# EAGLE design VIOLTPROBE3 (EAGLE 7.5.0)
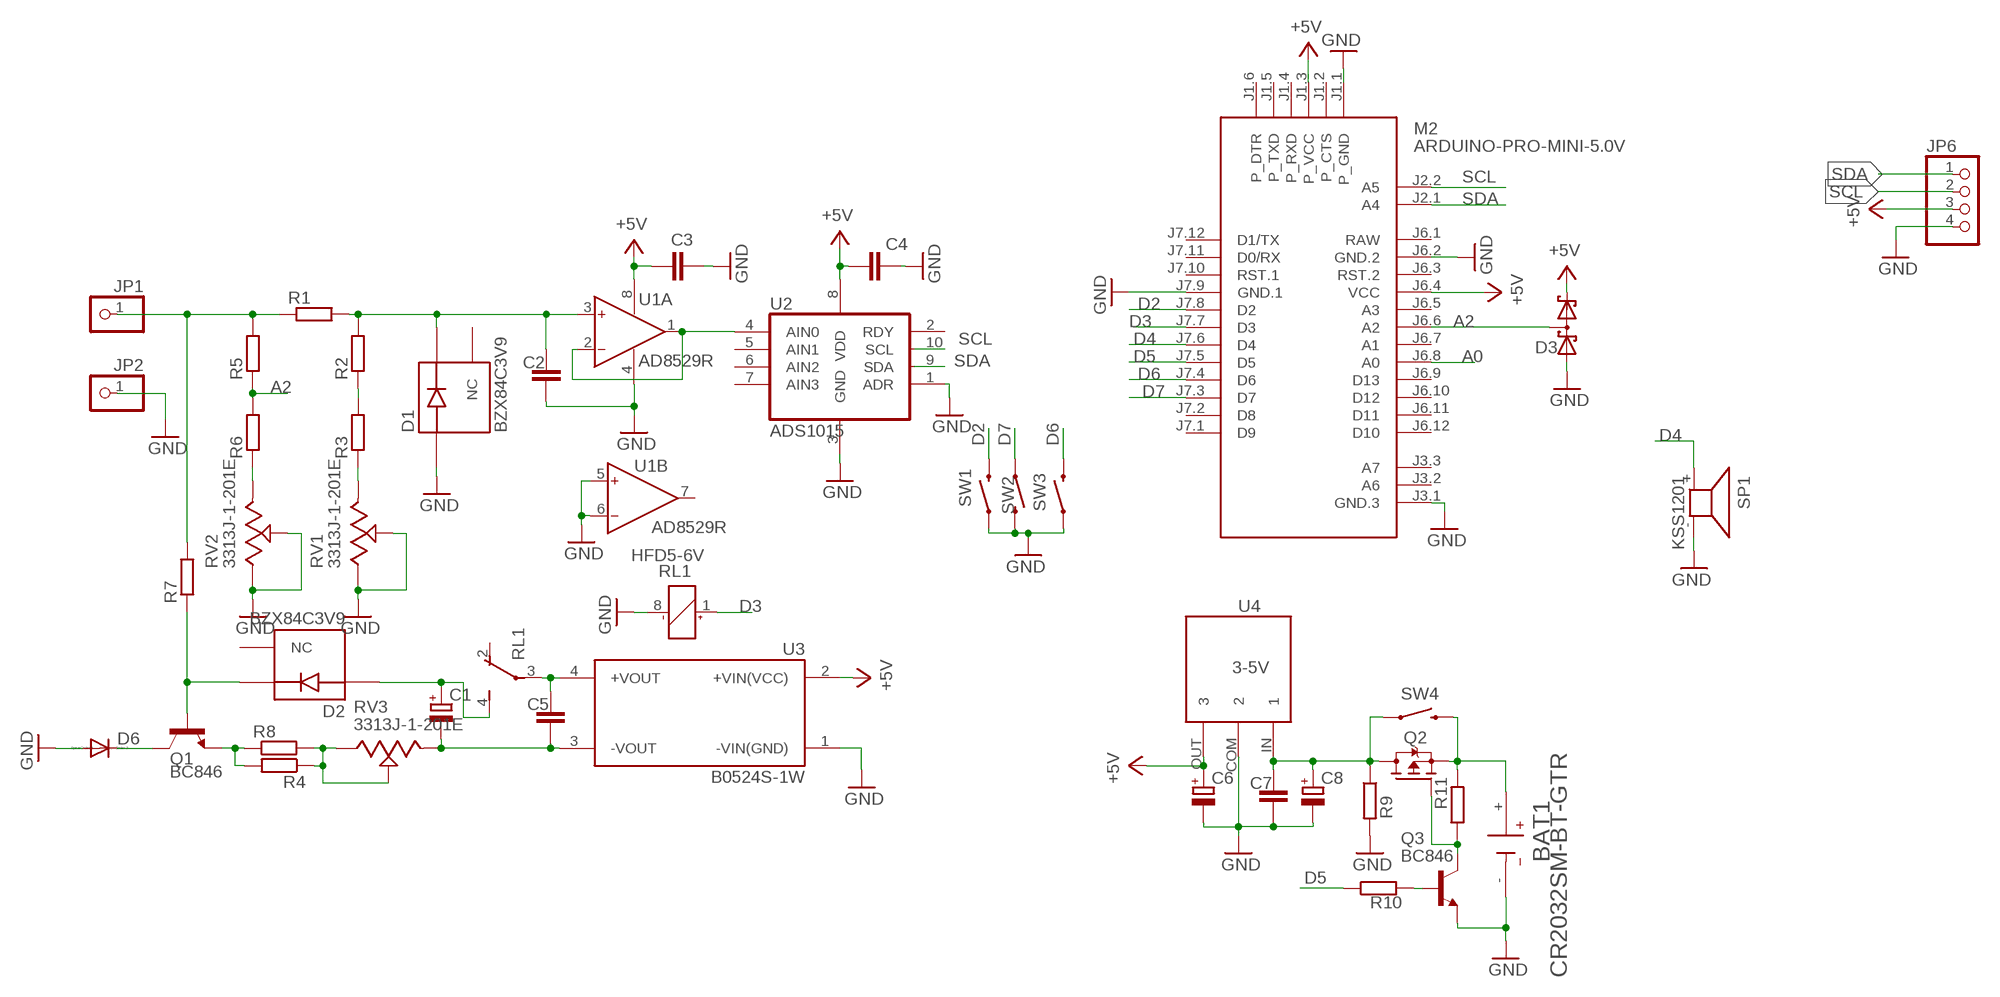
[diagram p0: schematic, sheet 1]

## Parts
BAT1  CR2032SM-BT-GTR  BU2032SM-BT-GTR  [BAT_BU2032SM-BT-GTR]
C1  CPOL-EUSMCA  [SMC_A]
C2  C-EUC0805  [C0805]
C3  C-EUC0805  [C0805]
C4  C-EUC0805  [C0805]
C5  C-EUC0805  [C0805]
C6  CPOL-EUSMCB  [SMC_B]
C7  C-EUC0805  [C0805]
C8  CPOL-EUSMCB  [SMC_B]
D1  BZX84C3V9  BZX84C15  [SOT95P237X112-3N]
D2  BZX84C3V9  BZX84C15  [SOT95P237X112-3N]
D3  BAT54S  [SOT23]
D6  CGRM4003-G  [SOD-123_MINI-SMA]
JP1  PINHD-1X1CB  [1X01-CLEANBIG]
JP2  PINHD-1X1CB  [1X01-CLEANBIG]
JP6  HEADER-1X4ROUND  [1X04_ROUND]
M2  ARDUINO-PRO-MINI-5.0V  [ARDUINO-PRO-MINI]
Q1  BC846  [SOT23]
Q2  STR2P3LLH6  [SOT23]
Q3  BC846  [SOT23]
R1  R-EU_R0603  [R0603]
R2  R-EU_R0603  [R0603]
R3  R-EU_R0603  [R0603]
R4  R-EU_R0603  [R0603]
R5  R-EU_R0603  [R0603]
R6  R-EU_R0603  [R0603]
R7  R-EU_R0603  [R0603]
R8  R-EU_R0603  [R0603]
R9  R-EU_R0603  [R0603]
R10  R-EU_R0603  [R0603]
R11  R-EU_R0603  [R0603]
RL1  HFD5-6V  G6J-2P-Y  [G6J-2P-Y]
RV1  3313J-1-201E  [TRIM_3313J-1-201E]
RV2  3313J-1-201E  [TRIM_3313J-1-201E]
RV3  3313J-1-201E  [TRIM_3313J-1-201E]
SP1  KSS1201  [KSS1201]
SW1  SWITCH-MOMENTARY-2SMD  [TACTILE-SWITCH-SMD]
SW2  SWITCH-MOMENTARY-2SMD  [TACTILE-SWITCH-SMD]
SW3  SWITCH-MOMENTARY-2SMD  [TACTILE-SWITCH-SMD]
SW4  SWITCH-MOMENTARY-2SMD  [TACTILE-SWITCH-SMD]
U1  AD8529R  [SO8]
U2  ADS1015  [ADS1015]
U3  B0524S-1W  TME_0505S  [CONV_TME_0505S]
U4  3-5V  [3-5V]

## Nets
+5V: C3.2 C4.2 C6.+ D3.2(C2) JP6.3 M2.J1.3(P_VCC) M2.J6.4(VCC) U1.8(P:V+) U2.8(VDD) U3.2(+VIN(VCC)) U4.OUT
A0: C7.2 C8.+ M2.J6.8(A0) Q2.1(D) R9.1 SW4.1 U4.IN
A2: D3.3(C1A2) M2.J6.6(A2) R5.1 R6.2
D2: M2.J7.8(D2) SW1.3
D3: M2.J7.7(D3) RL1.1(1:+)
D4: M2.J7.6(D4) SP1.+
D5: M2.J7.5(D5) R10.1
D6: M2.J7.4(D6) SW3.3
D7: M2.J7.3(D7) SW2.1
GND: BAT1.- C2.1 C3.1 C4.1 C6.- C7.1 C8.- D1.1(A) D3.1(A1) D6.A JP2.1 JP6.4 M2.J1.1(P_GND) M2.J3.1(GND.3) M2.J6.2(GND.2) M2.J7.9(GND.1) Q3.2(E) R9.2 RL1.8(1:-) RV1.1(CCW) RV1.2(WIPER) RV2.1(CCW) RV2.2(WIPER) SP1.- SW1.1 SW2.3 SW3.1 U1.4(P:V-) U1.5(B:IN+) U1.6(B:IN-) U2.1(ADR) U2.3(GND) U3.1(-VIN(GND)) U4.COM
N$1: JP1.1 R1.1 R5.2 R7.2
N$2: C2.2 D1.3(K) R1.2 R2.2 U1.3(A:IN+)
N$3: R2.1 R3.2
N$4: R3.1 RV1.3(CW)
N$5: U1.1(A:OUT) U1.2(A:IN-) U2.4(AIN0)
N$6: D2.3(K) Q1.1(B) R7.1
N$8: R6.1 RV2.3(CW)
N$9: Q1.2(E) R4.2 R8.1
N$10: D6.C Q1.3(C)
N$11: C1.- C5.1 RV3.3(CW) U3.3(-VOUT)
N$12: R4.1 R8.2 RV3.1(CCW) RV3.2(WIPER)
N$13: C5.2 RL1.3(2:P) U3.4(+VOUT)
N$14: C1.+ D2.1(A) RL1.4(2:S)
N$15: BAT1.+ Q2.3(S) R11.2 SW4.3
N$17: Q2.2(G) Q3.3(C) R11.1
N$18: Q3.1(B) R10.2
SCL: JP6.2 M2.J2.2(A5) U2.10(SCL)
SDA: JP6.1 M2.J2.1(A4) U2.9(SDA)
Unconnected: D1.2(NC) D2.2(NC) M2.J1.2(P_CTS) M2.J1.4(P_RXD) M2.J1.5(P_TXD) M2.J1.6(P_DTR) M2.J3.2(A6) M2.J3.3(A7) M2.J6.3(RST.2) M2.J6.5(A3) M2.J6.7(A1) M2.J6.9(D13) M2.J6.10(D12) M2.J6.11(D11) M2.J6.12(D10) M2.J7.1(D9) M2.J7.2(D8) M2.J7.10(RST.1) M2.J7.11(D0/RX) M2.J7.12(D1/TX) RL1.2(2:O) RL1.5(3:S) RL1.6(3:P) RL1.7(3:O) U1.7(B:OUT) U2.2(RDY) U2.5(AIN1) U2.6(AIN2) U2.7(AIN3)

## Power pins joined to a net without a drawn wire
RAW: M2.J6.1(RAW)

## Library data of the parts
BAT1 = BU2032SM-BT-GTR:BU2032SM-BT-GTR: Batt Holder Smt Coin 20mm Tape Check availability; AVAILABILITY: In Stock; CHECK_PRICES: https://www.snapeda.com/parts/BU2032SM-BT-GTR/MPD+%2528Memory+Protection+Devices%2529/view-part/?ref=eda; DESCRIPTION: Battery Holder (Open) Coin, 20.0mm 1 Cell SMD (SMT) Tab; MF: Memory Protection Devices; MP: BU2032SM-BT-GTR; PACKAGE: None; PRICE: None; SNAPEDA_LINK: https://www.snapeda.com/parts/BU2032SM-BT-GTR/MPD+%2528Memory+Protection+Devices%2529/view-part/?ref=snap
C1 C6 C8 = rcl:CPOL-EU: POLARIZED CAPACITOR, European symbol
C2-C5 C7 = rcl:C-EU: CAPACITOR, European symbol
D1 D2 = BZX84C15:BZX84C15: Check availability; AVAILABILITY: In Stock; CHECK_PRICES: https://www.snapeda.com/parts/BZX84C15/Onsemi/view-part/?ref=eda; DESCRIPTION: Zener Diode 15 V 225 mW ±6% Surface Mount SOT-23-3 (TO-236); MF: ON Semiconductor; MP: BZX84C15; PACKAGE: SOT-23-3 Fairchild Semiconductor; PRICE: None; SNAPEDA_LINK: https://www.snapeda.com/parts/BZX84C15/Onsemi/view-part/?ref=snap
D3 = diode:BAT54S: Schottky Diodes Pin connection corrected 2011-05-04 Source: Fairchild .. BAT54.pdf
D6 = diode:CGRM400*-G: Molded plasitc,JEDEC SOD-123/Mini SMA
JP1 JP2 = adafruit:PINHD-1X1: Pin header 1x1 for 0.1" spacing
JP6 = microbuilder:HEADER-1X4: PIN HEADER
M2 = diy-modules:ARDUINO-PRO-MINI-*: Arduino Pro Mini and compatible devices More details available here: https://www.arduino.cc/en/Main/ArduinoBoardProMini Click here to find device on ebay.com
Q1 Q3 = transistor:BC846: NPN TRANSISTOR
Q2 = transistor-fet:STR2P3LLH6
R1-R11 = rcl:R-EU_: RESISTOR, European symbol
RL1 = relay:G6J*-2?-Y: Surface-Mounting Signal Relay - G6J-Y 5.7 x 10.6 x 9 mm Source: http://www.omroncomponents.eu/ .. K125-E2-02-X.pdf; MF: OMRON COMPONENTS USA; MPN: G6J-2P-Y-DC12; OC_FARNELL: unknown; OC_NEWARK: 70J9830
RV1-RV3 = Trimmer_3x3:3313J-1-201E: Check availability; AVAILABILITY: In Stock; CHECK_PRICES: https://www.snapeda.com/parts/3313J-1-201E/Bourns/view-part/?ref=eda; DESCRIPTION: 3mm Sq, SMD, TRIMMER, Cermet, Single Turn, 200 ohms | Bourns 3313J-1-201E; MF: Bourns; MP: 3313J-1-201E; PACKAGE: SMD-3 Bourns; PRICE: None; SNAPEDA_LINK: https://www.snapeda.com/parts/3313J-1-201E/Bourns/view-part/?ref=snap
SP1 = buzzer:KSS1201: SPEAKER; OC_FARNELL: unknown; OC_NEWARK: unknown
SW1-SW4 = SparkFun-Electromechanical:SWITCH-MOMENTARY-2: Various NO switches- pushbuttons, reed, etc; PROD_ID: SWCH-08247
U1 = analog-devices:AD8529: 8 MHz Rail-to-Rail Operational Amplifiers Source: http://www.analog.com/static/imported-files/data_sheets/AD8519_8529.pdf; MF: ALTERA CORPORATION; MPN: AD8529ARZ; OC_FARNELL: unknown; OC_NEWARK: 59K6807
U2 = burr-brown:ADS1015: 12BIT I2C DAC
U3 = TME_0505S:TME_0505S: Check availability; AVAILABILITY: In Stock; CHECK_PRICES: https://www.snapeda.com/parts/TME%200505S/Traco+Power/view-part/?ref=eda; DESCRIPTION: 1 Watt DC/DC converter, industrial, ±10% input, unregulated, encapsulated, SIP-4 package; MF: Traco Power; MP: TME 0505S; PACKAGE: SIP-4 Traco Power; PRICE: None; SNAPEDA_LINK: https://www.snapeda.com/parts/TME%200505S/Traco+Power/view-part/?ref=snap
U4 = dc-dc-converter:3-5V

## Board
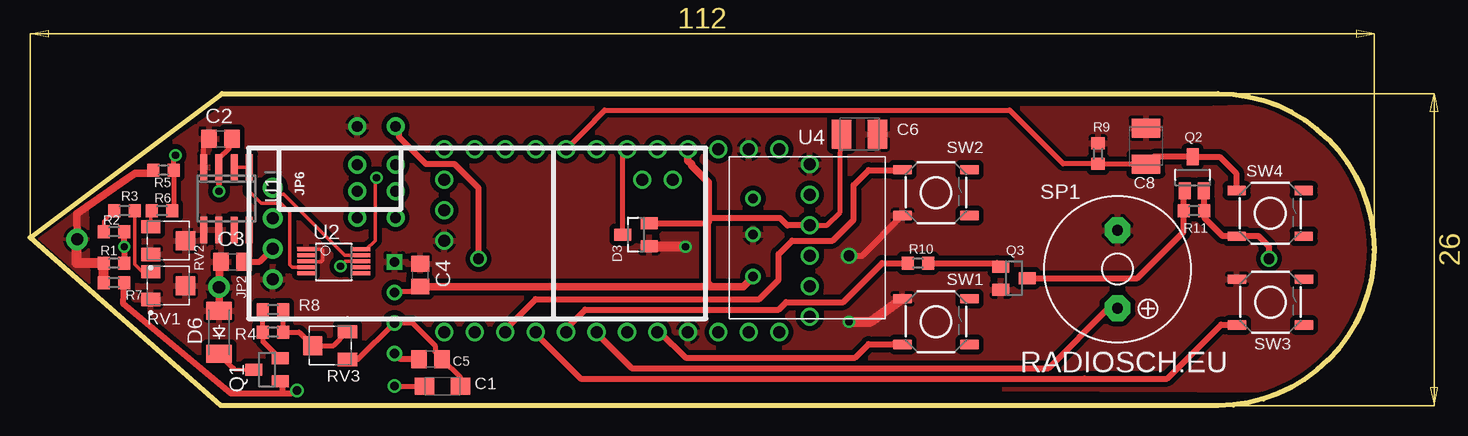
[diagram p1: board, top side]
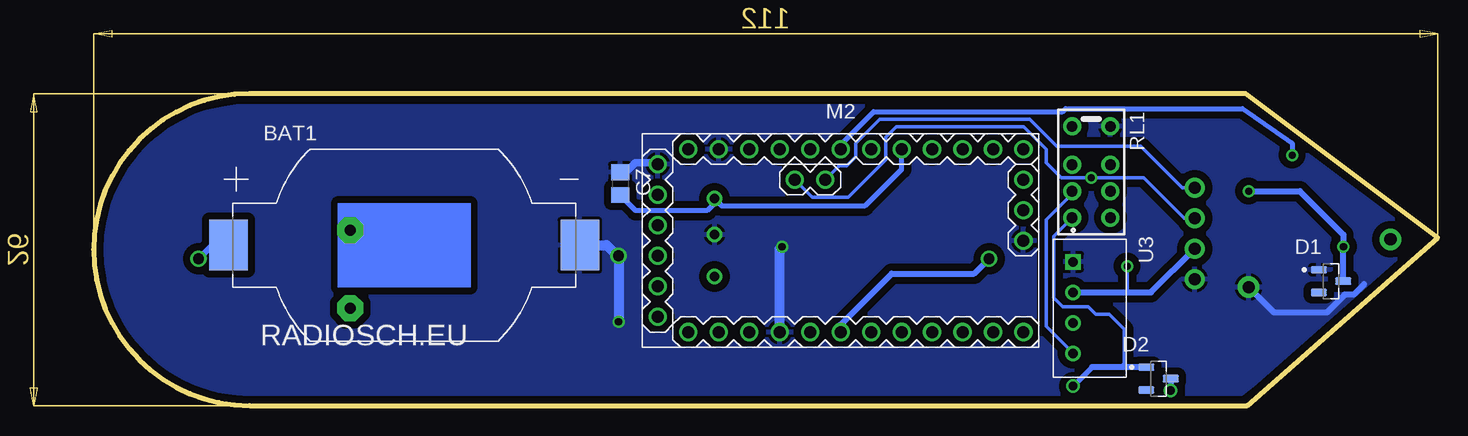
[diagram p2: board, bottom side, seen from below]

Size 117.3 x 31.3 mm. Coordinates in mm from the lower left corner, seen from the top.
Outline: 0,14 16,26 99,26 arc-180 99,0 15.88,0 0,14
Copper layers (1*16): Top 0.035mm / dielectric 1.5mm / Bottom 0.035mm
Design rules "default *": minimum track width 10mil, minimum drill 20mil, track to track 6mil, track to pad 6mil, pad to pad 6mil, via to via 6mil, smd to smd 6mil, copper to edge 6mil, drill to drill 6mil, minimum pad ring 10mil, minimum via ring 8mil, stop-mask expansion 4mil, vias tented up to drill 20mil, thermal gap 10mil

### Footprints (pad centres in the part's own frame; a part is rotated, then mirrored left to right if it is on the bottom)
BAT_BU2032SM-BT-GTR = smd 3.2 x 4.2: + -14.65,0; - 14.65,0
SMC_A = smd 1.6 x 1.4: + -1.5,0; - 1.5,0
C0805 = smd 1.3 x 1.5: 1 -0.95,0; 2 0.95,0
SMC_B = smd 1.6 x 2.4: + -1.5,0; - 1.5,0
SOT95P237X112-3N = smd 1.32 x 0.59: 1 -1.015,0.95; 2 -1.015,-0.95; 3 1.015,0
SOT23 = smd 1 x 1.4: 1 -0.95,-1.1; 2 0.95,-1.1; 3 0,1.1
SOD-123_MINI-SMA = smd 1.5 x 2.1: A 1.8,0; C -1.8,0
1X01-CLEANBIG = drill 1.016 pad 1.778: 1 0,0
1X04_ROUND = drill 1 pad 1.676: 1 -3.81,0; 2 -1.27,0; 3 1.27,0; 4 3.81,0
ARDUINO-PRO-MINI = drill 1: J1.1 -15.24,6.35; J1.2 -15.24,3.81; J1.3 -15.24,1.27; J1.4 -15.24,-1.27; J1.5 -15.24,-3.81; J1.6 -15.24,-6.35; J2.1 -1.27,5.08; J2.2 -3.81,5.08; J3.1 15.24,0; J3.2 15.24,2.54; J3.3 15.24,5.08; J6.1 -12.7,7.62; J6.2 -10.16,7.62; J6.3 -7.62,7.62; J6.4 -5.08,7.62; J6.5 -2.54,7.62; J6.6 0,7.62; J6.7 2.54,7.62; J6.8 5.08,7.62; J6.9 7.62,7.62; J6.10 10.16,7.62; J6.11 12.7,7.62; J6.12 15.24,7.62; J7.1 15.24,-7.62; J7.2 12.7,-7.62; J7.3 10.16,-7.62; J7.4 7.62,-7.62; J7.5 5.08,-7.62; J7.6 2.54,-7.62; J7.7 0,-7.62; J7.8 -2.54,-7.62; J7.9 -5.08,-7.62; J7.10 -7.62,-7.62; J7.11 -10.16,-7.62; J7.12 -12.7,-7.62
SOT23' = smd 1 x 1.4: 1 0,1.735; 2 -0.632,-1.1; 3 0.95,-1.1
R0603 = smd 1 x 1.1: 1 -0.85,0; 2 0.85,0
G6J-2P-Y = drill 0.9 pad 1.5: 1 -3.2,-1.6; 2 0,-1.6; 3 2.2,-1.6; 4 4.4,-1.6; 5 4.4,1.6; 6 2.2,1.6; 7 0,1.6; 8 -3.2,1.6
TRIM_3313J-1-201E = smd 1.1 x 1.6: 1 1.15,-1.45; 3 -1.15,-1.45 | smd 1.6 x 1.6: 2 0,1.45
KSS1201 = drill 0.914 pad 2.159 octagon: + 3.251,0; - -3.251,0
TACTILE-SWITCH-SMD = smd 1.524 x 0.762: 1 -2.794,1.905; 2 2.794,1.905; 3 -2.794,-1.905; 4 2.794,-1.905
SO8 = smd 0.6 x 2.2: 1 -1.905,-2.6; 2 -0.635,-2.6; 3 0.635,-2.6; 4 1.905,-2.6; 5 1.905,2.6; 6 0.635,2.6; 7 -0.635,2.6; 8 -1.905,2.6
ADS1015 = smd 0.3 x 1.5: 1 -1.905,-2.616; 2 -1.405,-2.616; 3 -0.905,-2.616; 4 -0.405,-2.616; 5 0.095,-2.616; 6 0.095,1.984; 7 -0.405,1.984; 8 -0.905,1.984; 9 -1.405,1.984; 10 -1.905,1.984
CONV_TME_0505S = drill 0.79 pad 1.19 square: 1 -3.85,0 | drill 0.79 pad 1.19: 2 -1.31,0; 3 1.23,0; 4 3.77,0
3-5V = drill 0.8: COM 0,-4; IN 0,-1; OUT 0,-7.5

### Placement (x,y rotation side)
BAT1  86.12,13.38 0 bottom
C1  34.38,1.62 0 top
C2  15.88,22.25 0 top
C3  16.88,12 0 top
C4  32.5,10.88 270 top
C5  33.38,3.88 180 top
C6  69.12,22.62 0 top
C7  68.12,18.5 270 bottom
C8  93,21.62 90 top
D1  8.88,10.38 0 bottom
D2  23.25,2.25 0 bottom
D3  50.5,14.25 90 top
D6  15.75,6.12 90 top
JP1  3.93,13.85 0 top
JP2  15.75,9.88 0 top
JP6  20.24,14.35 270 top
M2  49.75,13.75 0 bottom
Q1  19.75,3 90 top
Q2  STR2P3LLH6  [SOT23']  96.88,19 0 top
Q3  82,10.62 270 top
R1  7,11.88 0 top
R2  7,14.5 0 top
R3  7.88,16.25 180 top
R4  20.25,6.12 180 top
R5  11.12,19.62 180 top
R6  11,16.25 0 top
R7  7,10.25 180 top
R8  20.25,8 0 top
R9  89,21 90 top
R10  74,11.88 0 top
R11  97,16.25 0 top
RL1  28.86,20.07 270 bottom
RV1  11.5,10 270 top
RV2  11.5,13.75 270 top
RV3  25,5 90 top
SP1  90.62,11.38 270 top
SW1  75.5,7 0 top
SW2  75.5,17.75 0 top
SW3  103.38,8.62 0 top
SW4  103.35,16.02 0 top
U1  16.38,17.25 180 top
U2  25.62,11.12 270 top
U3  30.38,8.12 270 bottom
U4  60.25,18.25 0 top

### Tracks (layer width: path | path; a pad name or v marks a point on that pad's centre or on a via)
+5V  (via drill 0.6)
  Top 0.305: U2.8 26.28,12.03 v25.88,11.62
  Top 0.406: C4.2 32.17,9.93 31.75,9.5 30.44,9.5 U3.2 | M2.J1.3 66.39,15.02 67.5,16.12 67.5,20.88 C6.+
  Top 0.506: JP6.3 19.16,12 C3.2 18.28,12.46 U1.8 | 56.62,10.05 56.75,9.93 | D3.2 56.38,15.2 56.45,15.2 | M2.J1.3 63.1,15.02 62.5,15.62 56.5,15.62
  Top 0.61: C4.2 56.75,9.93 59.42,9.93 U4.OUT | M2.J6.4 54.83,20.42 55.12,20.12 55.12,20 56.5,18.62 56.5,15.62 56.5,15.32 56.38,15.2 | 56.45,15.2 56.45,10.22 56.62,10.05
  Bottom 0.305: v25.88,11.62 25.88,9.56 25.75,9.43
  Bottom 0.506: U3.2 25.75,9.43 23.89,9.43 JP6.3
A0
  Top 0.406: M2.J6.8 47.05,23.75 47.05,23.8 47.88,24.62 81.62,24.62 86.1,20.15 R9.1 92.97,20.15 C8.+
  Top 0.506: C8.+ 93.61,20.73 Q2.1 99.14,20.73 100.5,19.38 100.5,17.98 SW4.1
  Bottom 0.406: M2.J6.8 44.67,19.7 47.75,16.62 59.62,16.62 U4.IN 60.25,16.88 60.88,16.25 66.83,16.25 C7.2
A2  (via drill 0.6)
  Top 0.406: v12.12,20.88 11.97,20.73 R5.1 11.97,16.38 R6.2 | D3.3 49.4,21.02 M2.J6.6
  Bottom 0.406: 12.25,20.88 v12.12,20.88 12.12,21.88 16.25,24.75 31,24.75 31.25,24.5 47,24.5 49.62,21.88 49.62,21.5 M2.J6.6
D2
  Top 0.506: SW1.3 71.93,5.12 69.88,5.12 68.75,4 54.62,4 52.49,6.13 M2.J7.8
D3  (via drill 0.9)
  Top 0.506: v37.38,12.25 37.38,18.12 35.38,20.12 33,20.12 30.75,22.38 30.75,22.98 RL1.1
  Bottom 0.506: M2.J7.7 49.75,6.75 45.5,11 38.62,11 v37.38,12.25
D4
  Top 0.506: M2.J7.6 47.21,6.04 50.12,3.12 84.88,3.12 89.87,8.12 SP1.+
D5
  Top 0.506: M2.J7.5 44.67,6.42 46.25,8 62.38,8 63,8.62 67.75,8.62 71,11.88 R10.1
D6
  Top 0.5: 87.88,2.25 94.75,2.25 99.25,6.75 100.55,6.75 SW3.3
  Top 0.506: M2.J7.4 42.13,5.99 45.88,2.25 87.88,2.25
D7
  Top 0.506: M2.J7.3 39.59,6.34 42.12,8.88 60.75,8.88 62.38,10.5 62.38,12.62 63.5,13.75 66.88,13.75 68.62,15.5 68.62,18.38 69.88,19.62 72.68,19.62 SW2.1
GND  (via drill 0.6, 0.9)
  Top 0.305: U2.1 24.34,13.03 24.38,13 24.38,12.12 24.25,12 23.04,12 U2.3
  Top 0.406: U1.4 14.47,21.8 C2.1
  Top 0.506: v68.25,12.5 69.36,12.5 SW2.3
  Top 0.61: 15.57,7.75 D6.A JP2.1 15.75,11.82 C3.1
  Top 0.813: v54.62,13.25 51.65,13.25 D3.1 | v68.25,7 70.05,7 SW1.1
  Bottom 0.5: 6.12,10.12 7,9.25 7.75,9.25 9.25,7.75 13.62,7.75 JP2.1
  Bottom 0.506: C7.1 68.12,19.5 | 65.02,20.12 M2.J1.1 | BAT1.- 69.12,13.38 v68.25,12.5
  Bottom 0.61: 68.12,19.5 67.62,19.5 66.88,20.25 65.14,20.25 M2.J1.1
  Bottom 0.813: M2.J7.9 54.83,13.04 v54.62,13.25 | BAT1.- 69.25,13.38 68.25,12.38 v68.25,7
  pour Top (isolate 0.406, rank 2): 0.5,14.25 16,24.75 97.25,24.75 112.5,25.25 113.5,1.25 16,1.75
  pour Bottom (isolate 0.61): -0.12,13.88 16.12,25 99.12,25 113.38,24.75 113.38,1.38 99.88,0.88 16.38,1 0,13.88
N$1
  Top 0.406: 3.88,13 3.88,13.79 JP1.1
  Top 0.61: JP1.1 3.88,16 8,18.88 8.75,19.38 10.03,19.38 R5.2
  Top 0.813: 3.88,13 3.88,11.88 R1.1 R7.2
  pour Top: 0.75,13.88 4.62,16.75 4.75,16.88 4.88,10.25
N$2  (via drill 0.6)
  Top 0.406: U1.3 15.74,20.62 16.62,21.5 16.62,22.05 C2.2
  Top 0.506: R1.2 v7.85,13.25 R2.2 | U1.3 v15.74,17.88 v15.75,17.88
  Bottom 0.506: D1.3 v7.86,13.24 v7.85,13.25 7.85,14.25 11.47,17.88 v15.75,17.88
N$3
  Top 0.305: R2.1 6.15,15.38 R3.2
N$4
  Top 0.305: R3.1 8.72,11.78 9.25,11.25 9.95,11.25 RV1.3
N$5
  Top 0.305: U2.4 21.84,11.53 21.62,11.75 21.62,16.12 20.88,16.88 19.25,16.88 18.25,17.88 18.25,19.82 U1.1 U1.2
N$6  (via drill 0.7)
  Top 0.5: 21,1 21.75,1 22,1.25 v22.25,1.25 | 21,1 16.75,1 7.75,8.5 R7.1 | 21.02,1.88 21.02,1.03 21,1
  Top 0.506: 21.02,1.88 Q1.1
  Bottom 0.5: D2.3 22.23,1.27 v22.25,1.25
N$8
  Top 0.305: RV2.3 10.05,16.15 R6.1
N$9
  Top 0.406: 21.3,4.12 Q1.2 20.8,3.95 19.4,5.35 R4.2 R8.1
N$10
  Top 0.305: Q1.3 17.07,3 D6.C
  Top 0.406: 16.95,3.12 D6.C
N$11
  Top 0.406: U3.3 31.86,6.89 33.75,5 33.75,4.45 C5.1 | 34.38,3.82 C5.1 | 30.36,6.88 U3.3 | C1.- 35.88,2.32 C5.1 | RV3.3 27.33,3.85 U3.3
N$12
  Top 0.406: R4.1 21.1,7.25 | 21.1,7.25 R8.2 | 21.23,7.38 21.1,7.25 | 21.38,6.12 22.43,6.12 RV3.2 25.3,5 RV3.1
  Top 0.506: R4.1 21.38,6.12
N$13
  Top 0.506: C5.2 30.86,3.88 U3.4
  Bottom 0.305: RL1.3 30.46,17.66 32.62,15.5 32.62,6.62 30.77,4.77 30.77,4.75 U3.4
N$14  (via drill 0.7)
  Top 0.406: v30.38,1.62 C1.+
  Bottom 0.305: RL1.4 32,14.13 32,9 31.25,8.25 29.12,8.25 28.5,7.62 27.38,7.62 26.12,6.38 26.12,3.34
  Bottom 0.406: 28.8,3.2 v30.38,1.62
  Bottom 0.5: D2.1 26.25,3.2 | 26.25,3.2 28.8,3.2 | 26.12,3.34 26.12,3.32 26.25,3.2
N$15  (via drill 0.9)
  Top 0.506: 100.57,14.12 102.38,14.12 103.25,13.25 v103.25,12.25 | 100.57,14.12 SW4.3 | Q2.3 97.85,17.88 R11.2 97.88,16.23 97.88,15.62 99.38,14.12 100.57,14.12
  Bottom 0.506: BAT1.+ 100.78,13.47 100.62,13.62 101.88,13.62 v103.25,12.25
N$17
  Top 0.506: Q3.3 92.25,10.62 96.12,14.5 96.12,16.23 R11.1 96.15,17.81 Q2.2
N$18
  Top 0.506: R10.2 80.6,11.88 Q3.1
SCL  (via drill 0.6)
  Top 0.305: U2.10 28.03,13.03 28.75,13.75 28.75,18.88 v28.88,19
  Bottom 0.305: JP6.2 21.12,15.62 24.5,19 v28.88,19 31.38,19 32.62,20.25 32.62,21.38 34.5,23.25 45.12,23.25 46,22.38 46,20.5 46.12,20.38 46.5,20 49.12,17.38 52.1,17.38 M2.J2.2
SDA
  Top 0.305: U2.9 26.22,12.53 21.12,17.62 20.77,17.62 JP6.1
  Bottom 0.305: JP6.1 21.29,18.16 24.75,21.62 31.75,21.62 34,23.88 46.5,23.88 48.5,21.88 48.5,20.75 49.25,20 49.85,20 M2.J2.1

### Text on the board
tPlace: RADIOSCH.EU
bPlace: RADIOSCH.EU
